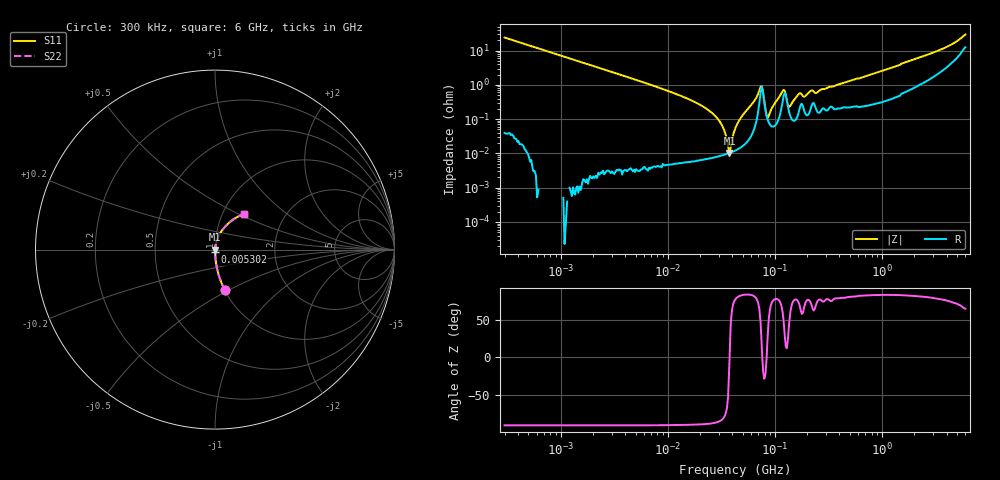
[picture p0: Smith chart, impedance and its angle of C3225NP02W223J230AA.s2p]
! S-Parameter Data Generated by TDK Corporation
! Copyright(C) 2024 TDK Corporation.
! All Rights Reserved.
! TDK P/N: C3225NP02W223J230AA (Multilayer Ceramic Chip Capacitor)
! Property: C=22nF
! Size(LxWxT): 3.2x2.5x2.3mm
! Model Type: s2p (Touchstone File Format Version 1.0)
! Frequency: DC=Yes Start=0.3MHz Stop=6000MHz 402points Log-sweep
! Model Generated on May 28, 2024
! Terms and conditions regarding TDK Simulation Models:
! 1)This simulation model is being provided solely for informational
!  purposes. Please refer to the specifications of the products in
!  terms of detailed characteristics of such products.
! 2)In no event shall TDK Corporation of any of its subsidiaries be
!  liable for any loss or damage arising, directly or indirectly,
!  from any information contained in this simulation model, including,
!  but not limited to loss or damages arising from any inaccuracies,
!  omissions or errors in connection with such information.
! 3)Any and all copyrights on this simulation model are owned by
!  TDK Corporation.  Duplication or redistribution of this simulation
!  model without prior written permission from TDK Corporation
!  is prohibited.
! 4)This simulation model is subject to any modification or change
!  without any prior notice.
! 5)Neither TDK Corporation nor any of its subsidiaries shall make any
!  warranty, express or implied, including but not limited to the
!  correctness, implied warranties of merchantability and fitness for
!  a particular purpose with respect to this simulation models.
! 6)The use of this simulation model shall be deemed to have consented
!  to the terms and conditions hereof.
! Port Assignments:
!  1 ---| |--- 2
! Applicable Conditions:
!  Temperature = 25 degC
!  DC Bias Voltage = 0 V
!  Small Signal Operation
# Hz S MA R 50
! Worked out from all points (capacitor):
!   401 points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, 300 kHz to 6 GHz, reference 50 ohm
!   read as one part in series: C = 22.1 nF near 317.3 kHz
!   lowest |Z| = 10.4 mohm at 37.62 MHz (marker M1)
!   series resonance near 37.74 MHz, so ESL is about 800 pH
!   S11 on the Smith chart (normalised r, x): 300 kHz: 1.00, -0.48; 5.302 MHz: 1.00, -0.03; 6 GHz: 1.25, +0.53
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300000  0.2333 -76.4  0.972 13.5  0.972 13.5  0.2333 -76.4
1586297  0.04523 -87.4  0.999 2.6  0.999 2.6  0.04523 -87.4
5301759  0.0133 -89.1  0.9999 0.8  0.9999 0.8  0.0133 -89.1
8158352  0.008414 -89.2  0.9999 0.5  0.9999 0.5  0.008414 -89.2
2.474969e7  0.001701 -87.5  0.9999 0.1  0.9999 0.1  0.001701 -87.5
3.109046e7  0.0007828 -83.7  0.9999 0.0  0.9999 0.0  0.0007828 -83.7
3.762394e7  0.0001037 -6.9  0.9999 0.0  0.9999 0.0  0.0001037 -6.9
3.973252e7  0.0002411 62.8  0.9999 -0.0  0.9999 -0.0  0.0002411 62.8
4.28954e7  0.0005584 77.3  0.9999 -0.0  0.9999 -0.0  0.0005584 77.3
4.922114e7  0.001215 82.5  0.9998 -0.1  0.9998 -0.1  0.001215 82.5
7.36264e7  0.008805 45.0  0.9938 -0.4  0.9938 -0.4  0.008805 45.0
7.764022e7  0.00597 -18.7  0.9943 0.1  0.9943 0.1  0.00597 -18.7
8.366094e7  0.00125 -1.4  0.9988 0.0  0.9988 0.0  0.00125 -1.4
8.767476e7  0.001261 50.8  0.9992 -0.1  0.9992 -0.1  0.001261 50.8
1.181956e8  0.006528 59.2  0.9967 -0.3  0.9967 -0.3  0.006528 59.2
1.401524e8  0.00253 62.4  0.9988 -0.1  0.9988 -0.1  0.00253 62.4
1.668943e8  0.00535 72.4  0.9984 -0.3  0.9984 -0.3  0.00535 72.4
1.933677e8  0.004767 72.7  0.9986 -0.3  0.9986 -0.3  0.004767 72.7
2.249926e8  0.006818 64.5  0.9971 -0.4  0.9971 -0.4  0.006818 64.5
1.174439e9  0.02995 81.2  0.9959 -1.7  0.9959 -1.7  0.02995 81.2
3.696743e9  0.1104 70.4  0.9686 -6.2  0.9686 -6.2  0.1104 70.4
6e9  0.2552 51.4  0.8642 -13.3  0.8642 -13.3  0.2552 51.4
